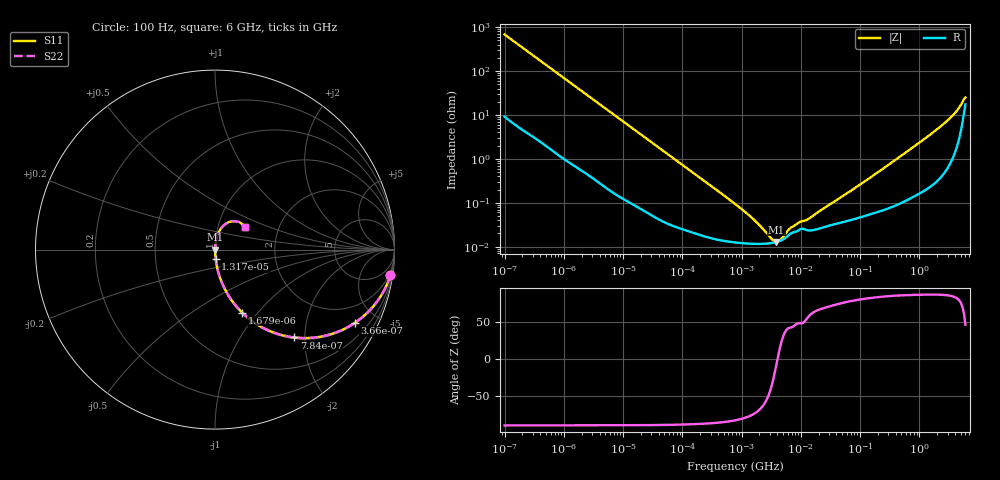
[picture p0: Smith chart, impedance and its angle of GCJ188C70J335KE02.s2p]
!Murata Part Number: GCJ188C70J335KE02
!These Parameters are Measured in Series Mode Connection
!Data Generated on Mar 13, 2026
!  o--ll--o
!Port1  Port2
!  o------o
!Operation Temp=25[degC], DC Bias Voltage=0[V]
!Freq. Start=100[Hz] Stop=6[GHz] 401[Steps]
# Hz S RI R 50
!Freq.(Hz) S11(Real) S11(Imag) S21(Real) S21(Imag) S12(Real) S12(Imag) S22(Real) S22(Imag)
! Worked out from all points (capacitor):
!   401 points, 100 Hz to 6 GHz, reference 50 ohm
!   read as one part in series: C = 2.32 uF near 109 Hz
!   lowest |Z| = 12.8 mohm at 3.882 MHz (marker M1)
!   series resonance near 4.05 MHz, so ESL is about 670 pH
!   S11 on the Smith chart (normalised r, x): 100 Hz: 1, -14; 366 Hz: 1.05, -3.77; 784 Hz: 1.03, -1.77; 1.679 kHz: 1.01, -0.83; 13.17 kHz: 1.00, -0.11; 6 GHz: 1.35, +0.36
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100  0.9772 -0.1426  0.0228 0.1426  0.0228 0.1426  0.9772 -0.1426
205  0.9156 -0.2715  0.0844 0.2715  0.0844 0.2715  0.9156 -0.2715
366  0.7774 -0.409  0.2226 0.409  0.2226 0.409  0.7774 -0.409
548  0.6141 -0.4798  0.3859 0.4798  0.3859 0.4798  0.6141 -0.4798
784  0.4414 -0.4895  0.5586 0.4895  0.5586 0.4895  0.4414 -0.4895
1174  0.2644 -0.4339  0.7356 0.4339  0.7356 0.4339  0.2644 -0.4339
1679  0.152 -0.3515  0.848 0.3515  0.848 0.3515  0.152 -0.3515
2008  0.1125 -0.3084  0.8875 0.3084  0.8875 0.3084  0.1125 -0.3084
4702  0.0244 -0.1465  0.9756 0.1465  0.9756 0.1465  0.0244 -0.1465
13169  0.00392 -0.054  0.9961 0.054  0.9961 0.054  0.00392 -0.054
40335  0.000735 -0.0179  0.9993 0.0179  0.9993 0.0179  0.000735 -0.0179
774597  0.000125 -0.000935  0.9999 0.000935  0.9999 0.000935  0.000125 -0.000935
1658239  0.000116 -0.000382  0.9999 0.000382  0.9999 0.000382  0.000116 -0.000382
3245845  0.000121 -8.47e-05  0.9999 8.47e-05  0.9999 8.47e-05  0.000121 -8.47e-05
3882480  0.000127 -1.61e-05  0.9999 1.61e-05  0.9999 1.61e-05  0.000127 -1.61e-05
4643984  0.000138 5.27e-05  0.9999 -5.27e-05  0.9999 -5.27e-05  0.000138 5.27e-05
6948629  0.000204 0.000185  0.9998 -0.000185  0.9998 -0.000185  0.000204 0.000185
1.555665e7  0.000235 0.00043  0.9998 -0.00043  0.9998 -0.00043  0.000235 0.00043
3.124326e8  0.000813 0.00751  0.9992 -0.00751  0.9992 -0.00751  0.000813 0.00751
2.450438e9  0.00759 0.0584  0.9924 -0.0584  0.9924 -0.0584  0.00759 0.0584
4.385646e9  0.0348 0.1202  0.9652 -0.1202  0.9652 -0.1202  0.0348 0.1202
6e9  0.1683 0.1272  0.8317 -0.1272  0.8317 -0.1272  0.1683 0.1272
